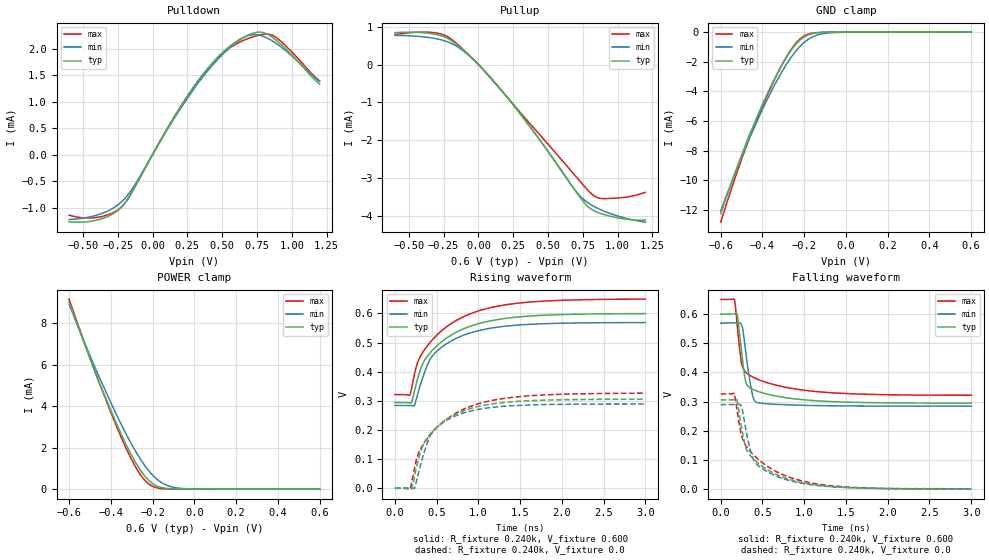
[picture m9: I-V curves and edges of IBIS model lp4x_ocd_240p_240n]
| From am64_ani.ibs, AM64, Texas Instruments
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|   Model lp4x_ocd_240p_240n
[Model] lp4x_ocd_240p_240n
Model_type I/O
Polarity   Non-Inverting
Enable   Active-High
Vinl =  0.0V
Vinh =  0.900V
Vmeas =  0.600V
C_comp   2.927pF   2.703pF   3.163pF
[Model Spec]
Vinh   0.900V   0.900V   0.900V
Vinl   0.0V   0.0V   0.0V
Vmeas   0.600V   NA   NA
[Temperature Range]   25.000   0.125k   -40.000
[Voltage Range]   0.600V   0.570V   0.650V
[Pullup Reference]   0.600V   0.570V   0.650V
[Pulldown Reference]   0.0V   0.0V   0.0V
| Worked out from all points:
|   slope of the pulldown table from 0 to 0.09 V, typ, clamps not added: 215 ohm
|   slope of the pullup table from 0 to 0.09 V, typ, clamps not added: 251 ohm
|   GND clamp passes 1 mA (typ) near -0.25 V on its own axis
|   POWER clamp passes 1 mA (typ) near -0.26 V on its own axis
|   rising waveform, R_fixture 0.240k, V_fixture 0.600: 20-80 % time 502ps typ, 425ps min, 554ps max; typ from 0.295 V to 0.599 V
|   rising waveform, R_fixture 0.240k, V_fixture 0.0: 20-80 % time 415ps typ, 324ps min, 517ps max; typ from 0 V to 0.306 V
|   falling waveform, R_fixture 0.240k, V_fixture 0.600: 20-80 % time 95.1ps typ, 85.9ps min, 174ps max; typ from 0.599 V to 0.295 V
|   falling waveform, R_fixture 0.240k, V_fixture 0.0: 20-80 % time 362ps typ, 278ps min, 432ps max; typ from 0.306 V to 0 V
[Pulldown]
|Voltage   I(typ)   I(min)   I(max)
-600mV    -1.271mA   -1.226mA   -1.144mA
-392mV    -1.233mA   -1.137mA   -1.183mA
-221mV    -984.9uA   -887.4uA   -982.9uA
-126mV    -608.1uA   -567.5uA   -606.4uA
120mV     553.9uA    533.1uA    552.7uA
309mV     1.328mA    1.286mA    1.326mA
480mV     1.869mA    1.83mA     1.853mA
651mV     2.213mA    2.204mA    2.155mA
764mV     2.314mA    2.258mA    2.256mA
859mV     2.217mA    2.15mA     2.256mA
954mV     2.004mA    1.969mA    2.061mA
1.2V      1.33mA     1.38mA     1.393mA
[Pullup]
|Voltage   I(typ)   I(min)   I(max)
-600mV    845.1uA    771.9uA    794.5uA
-411mV    846.4uA    738.5uA    858.9uA
-278mV    772.7uA    663.3uA    816.3uA
-202mV    652.7uA    571.6uA    692.4uA
-107mV    376.1uA    357.2uA    390.7uA
44.21mV   -171.8uA   -170.3uA   -175.6uA
234mV     -994.2uA   -986.8uA   -980.8uA
707mV     -3.392mA   -3.382mA   -2.991mA
783mV     -3.744mA   -3.647mA   -3.31mA
840mV     -3.888mA   -3.773mA   -3.498mA
1.011V    -4.066mA   -4.019mA   -3.529mA
1.2V      -4.12mA    -4.173mA   -3.383mA
[GND_clamp]
|Voltage   I(typ)   I(min)   I(max)
-600mV    -12.26mA   -12.07mA   -12.83mA
-535mV    -9.631mA   -9.657mA   -9.999mA
-483mV    -7.674mA   -7.84mA    -7.926mA
-457mV    -6.749mA   -6.974mA   -6.957mA
-378mV    -4.198mA   -4.571mA   -4.306mA
-326mV    -2.706mA   -3.156mA   -2.747mA
-287mV    -1.735mA   -2.22mA    -1.722mA
-248mV    -949.8uA   -1.424mA   -887.8uA
-209mV    -414uA     -806.5uA   -336.6uA
-157mV    -95.46uA   -302uA     -61.62uA
-78.26mV  -9.099uA   -53.02uA   -8.176uA
600mV     0A         0A         0A
[POWER_clamp]
|Voltage   I(typ)   I(min)   I(max)
-600mV    9.037mA    8.928mA    9.175mA
-457mV    5.197mA    5.441mA    5.166mA
-352mV    2.698mA    3.164mA    2.544mA
-313mV    1.878mA    2.4mA      1.683mA
-274mV    1.164mA    1.707mA    946.8uA
-248mV    770.5uA    1.297mA    560.3uA
-222mV    461.8uA    938.4uA    283.8uA
-196mV    246uA      638.9uA    120.5uA
-157mV    79.32uA    316.3uA    23.5uA
-117mV    22.66uA    136.3uA    6.085uA
-78.26mV  6.703uA    54.43uA    1.893uA
600mV     0A         0A         0A
[Ramp]
| variable   typ   min   max
dV/dt_r   0.183/0.416n   0.173/0.324n   0.196/0.523n
dV/dt_f   0.183/94.936p   0.171/85.592p   0.197/0.174n
R_load = 0.240k
[Rising Waveform]
R_fixture= 0.240k
V_fixture= 0.600
V_fixture_min= 0.570
V_fixture_max= 0.650
|time   V(typ)   V(min)   V(max)
0s        294.7mV    284.6mV    321.7mV
176ps     293.7mV    284.4mV    319.6mV
201ps     295.9mV    283.8mV    345.2mV
233ps     332.4mV    283.9mV    388.7mV
328ps     425.1mV    375.5mV    464.3mV
448ps     473.5mV    454.1mV    509.5mV
642ps     520.1mV    500.3mV    559.1mV
908ps     556.8mV    533.7mV    599.5mV
1.619ns   591.3mV    562.9mV    639.2mV
3ns       599.5mV    568.7mV    649.4mV
[Rising Waveform]
R_fixture= 0.240k
V_fixture= 0.0
V_fixture_min= 0.0
V_fixture_max= 0.0
|time   V(typ)   V(min)   V(max)
0s        471.3uV    1.984mV    519.6uV
179ps     -780.9uV   1.723mV    -2.098mV
201ps     -810.9uV   1.195mV    20.38mV
234ps     40.48mV    291.3uV    67.05mV
327ps     142.3mV    101.3mV    145.3mV
439ps     191.8mV    188.6mV    189.4mV
629ps     238.6mV    235.1mV    239.5mV
897ps     273.4mV    264.7mV    280.5mV
1.569ns   300.3mV    285.9mV    316.8mV
3ns       305.9mV    289.7mV    326.5mV
[Falling Waveform]
R_fixture= 0.240k
V_fixture= 0.600
V_fixture_min= 0.570
V_fixture_max= 0.650
|time   V(typ)   V(min)   V(max)
0s        599.5mV    568.7mV    649.4mV
164ps     600.6mV    568.8mV    648.4mV
202ps     590.7mV    569.6mV    548.4mV
249ps     470mV      563.7mV    430.8mV
268ps     424.8mV    541.7mV    412.8mV
306ps     362.3mV    454.3mV    399mV
375ps     343.1mV    330mV      385.5mV
430ps     336.5mV    297.3mV    377.9mV
1.258ns   301mV      285.9mV    331.7mV
3ns       294.7mV    284.4mV    321.7mV
[Falling Waveform]
R_fixture= 0.240k
V_fixture= 0.0
V_fixture_min= 0.0
V_fixture_max= 0.0
|time   V(typ)   V(min)   V(max)
0s        305.9mV    289.6mV    326.4mV
162ps     306.9mV    289.6mV    326.9mV
195ps     305mV      290.5mV    271.7mV
237ps     231.1mV    289.1mV    199.8mV
258ps     196.6mV    275.2mV    174.7mV
307ps     136.8mV    195.1mV    146.7mV
409ps     99.32mV    92.74mV    113.1mV
790ps     36.79mV    32.51mV    44.75mV
1.466ns   6.545mV    6.517mV    8.74mV
3ns       456.9uV    1.919mV    504uV
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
